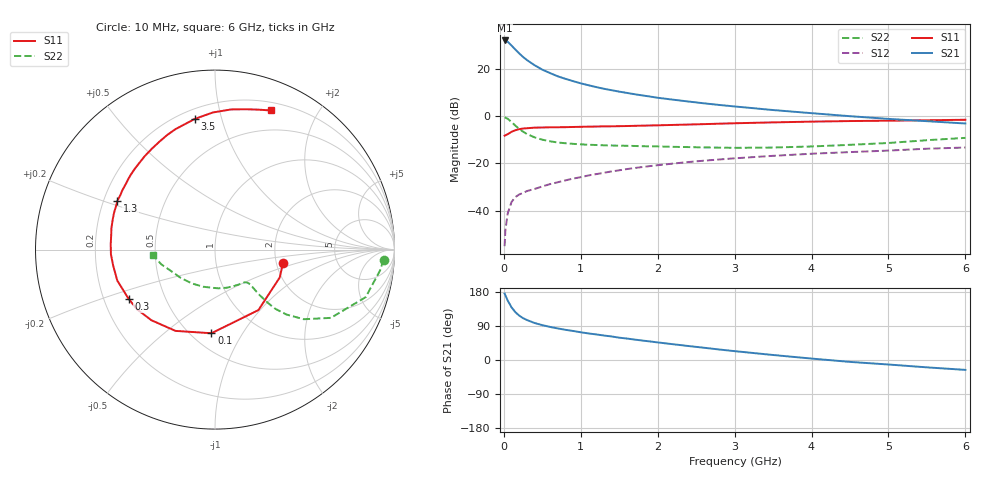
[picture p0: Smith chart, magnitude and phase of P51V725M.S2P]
! SIEMENS Small Signal Semiconductors
! BFP183
! Si NPN RF Bipolar Junction Transistor in SOT143
! VCE = 1.75 V  IC = 25 mA
! Common Emitter S-Parameters:  March  1996
# GHz  S  MA  R  50
!  f  S11  S21  S12  S22
! GHz  MAG  ANG  MAG  ANG  MAG  ANG  MAG  ANG
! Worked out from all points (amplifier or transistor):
!   36 points, 10 MHz to 6 GHz, reference 50 ohm
!   highest |S21| = 31.9 dB at 10 MHz (marker M1)
!   |S21| within 3 dB of that: start of sweep to 125.1 MHz
!   unconditionally stable (mu >= 1): 602.2 MHz to 5.825 GHz
!   at 250 MHz: K = 0.61, MSG = 28.7 dB, |S12| = -32.4 dB
!   at 1.4 GHz: K = 1.22, MAG = 14.3 dB, |S12| = -23.4 dB
!   at 6 GHz: K = 0.98, MSG = 5.1 dB, |S12| = -13.3 dB
!   S11 on the Smith chart (normalised r, x): 10 MHz: 2.17, -0.39; 100 MHz: 0.62, -0.74; 300 MHz: 0.31, -0.24; 1.3 GHz: 0.26, +0.22; 3.5 GHz: 0.26, +0.82; 6 GHz: 0.28, +1.45
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0.01  0.3861 -11.5  39.44 175.3  0.0018 81.5  0.9408 -3.4
0.02  0.3927 -23.3  39.14 170.7  0.0039 78.5  0.9269 -7.2
0.05  0.4148 -54.3  37.01 156.9  0.0088 73.2  0.8804 -17.5
0.1  0.4664 -92.4  30.8 139.0  0.0154 59.8  0.7494 -30.5
0.15  0.5035 -115.9  25.34 126.2  0.0196 53.0  0.6287 -38.1
0.2  0.5296 -132.0  21.01 117.1  0.0222 50.4  0.537 -42.3
0.25  0.547 -142.5  17.67 110.4  0.0239 49.1  0.4694 -44.5
0.3  0.554 -150.4  15.22 105.5  0.0262 48.9  0.4188 -45.2
0.4  0.5711 -162.4  11.83 97.6  0.029 49.1  0.3557 -45.6
0.5  0.5745 -171.2  9.555 92.0  0.0328 50.4  0.3179 -45.3
0.6  0.5804 -177.4  8.091 87.3  0.0367 52.2  0.2938 -44.9
0.7  0.5817 177.1  6.92 83.3  0.0401 53.7  0.2777 -44.8
0.8  0.5838 172.3  6.122 79.7  0.044 54.6  0.2673 -45.0
1.1  0.5988 159.9  4.477 70.1  0.0559 55.7  0.2486 -47.3
1.3  0.6078 153.4  3.775 64.6  0.0637 55.6  0.2421 -49.9
1.7  0.6234 140.6  2.893 53.9  0.0802 54.0  0.2342 -56.9
2.2  0.651 127.1  2.22 41.6  0.0995 50.1  0.2244 -68.2
2.8  0.6916 112.7  1.718 27.7  0.1215 44.7  0.2165 -85.0
3.5  0.7367 98.8  1.342 13.2  0.145 38.5  0.2171 -107.6
4.5  0.7859 83.5  0.995 -5.0  0.174 29.0  0.2477 -140.5
5.5  0.8163 72.8  0.781 -19.4  0.205 20.8  0.31 -164.6
6  0.8365 67.9  0.698 -26.1  0.2174 16.0  0.3471 -174.8
